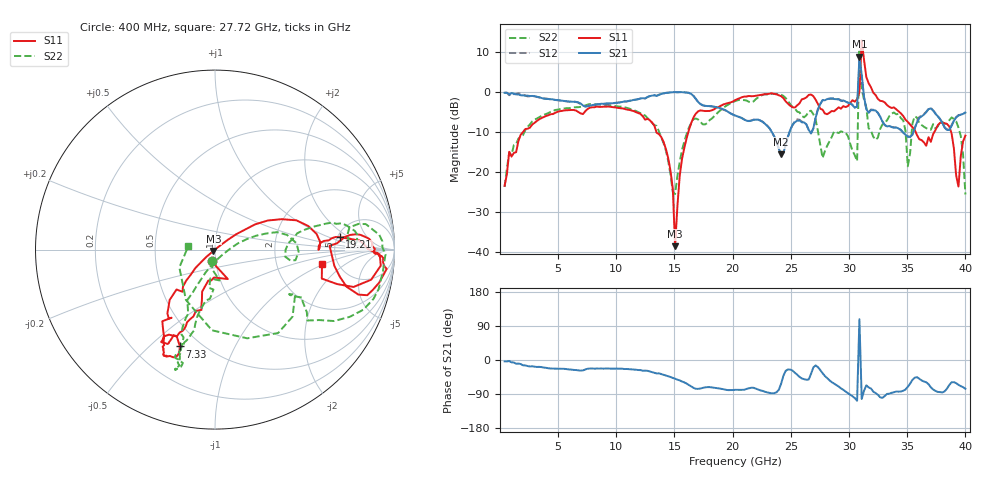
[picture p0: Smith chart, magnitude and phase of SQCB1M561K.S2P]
! Network Analyzer HP8722ES.07.66: Jul 25, 2000 Serial No. US39175408
! 27 Oct 2004  14:39:47
! Frequency  S11  S21  S12  S22
# HZ  S  DB R  50
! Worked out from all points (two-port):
!   201 points, 400 MHz to 40 GHz, reference 50 ohm
!   highest |S21| = 8.84 dB at 30.89 GHz (marker M1); lowest = -15.6 dB at 24.16 GHz (marker M2)
!   |S21| within 3 dB of the highest: 30.84 GHz to 31.02 GHz (177.7 MHz wide, 0.574 % of centre)
!   lowest |S11| = -38.5 dB at 15.05 GHz (marker M3), VSWR 1.02, Z = 49.1 - j0.739 ohm
!   |S11| at or under -10 dB: start of sweep to 1.987 GHz; 13.45 GHz to 16.19 GHz (2.747 GHz wide, 18.5 % of centre); 35.72 GHz to 37.34 GHz (1.612 GHz wide, 4.41 % of centre)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
!   |S22| runs from -25.6 to 10.7 dB; largest |S21 - S12| = 1.1
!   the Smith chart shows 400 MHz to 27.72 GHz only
!   S11 on the Smith chart (normalised r, x): 400 MHz: 0.95, -0.12; 7.33 GHz: 0.39, -0.63; 19.21 GHz: 5.23, +1.43; 27.72 GHz: 3.78, -0.92
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4e8  -23.42 -106.7  -0.21 -3.5  -0.16 -3.1  -23.75 -104.7
7.132e9  -5.53 -113.7  -3.38 -27.5  -3.46 -28.5  -3.65 -105.8
7.33e9  -4.83 -109.9  -3.65 -25.1  -3.61 -26.4  -3.36 -106.2
1.3666e10  -10.56 -127.6  -0.73 -35.2  -0.68 -35.3  -9.89 -118.8
1.4656e10  -19.69 -137.9  -0.14 -44.8  -0.11 -45.6  -20.67 -103.5
1.5052e10  -38.54 -140.5  -0.03 -49.3  -0.05 -50.0  -25.50 -26.4
1.6438e10  -7.80 24.6  -0.50 -69.4  -0.52 -70.4  -7.75 11.5
1.921e10  -3.12 5.7  -4.35 -77.1  -4.45 -77.7  -3.98 13.2
2.02e10  -2.06 6.2  -5.85 -78.7  -5.91 -79.4  -2.31 8.9
2.416e10  -1.05 -16.7  -15.58 -63.0  -15.59 -63.9  -0.68 -17.2
2.6932e10  -1.05 -10.9  -9.13 -19.6  -9.16 -19.9  -5.58 -70.1
2.7724e10  -4.42 -7.4  -2.08 -34.8  -2.06 -34.0  -16.50 172.3
3.0694e10  -1.79 0.9  -3.69 -107.6  -3.66 -107.7  -17.29 139.4
3.0892e10  -0.11 -72.6  8.84 107.6  5.42 93.8  10.69 3.6
3.109e10  12.87 -28.0  4.28 -102.9  4.09 -103.3  0.75 -160.9
3.1288e10  8.03 -40.5  -1.22 -81.2  -1.36 -81.5  -1.93 -118.2
3.1684e10  2.19 -54.5  -5.24 -72.3  -5.13 -74.5  -9.06 -127.3
3.3466e10  -3.74 -100.9  -8.51 -88.9  -8.49 -89.9  -6.03 167.5
3.505e10  -7.49 -166.3  -11.20 -70.8  -11.08 -70.9  -18.58 58.8
3.901e10  -14.05 19.0  -7.22 -58.4  -7.14 -58.6  -6.75 139.5
3.9406e10  -23.64 -136.2  -5.90 -65.5  -5.80 -66.1  -8.90 113.5
4e10  -10.92 133.0  -5.16 -76.0  -5.12 -76.5  -25.61 16.0
